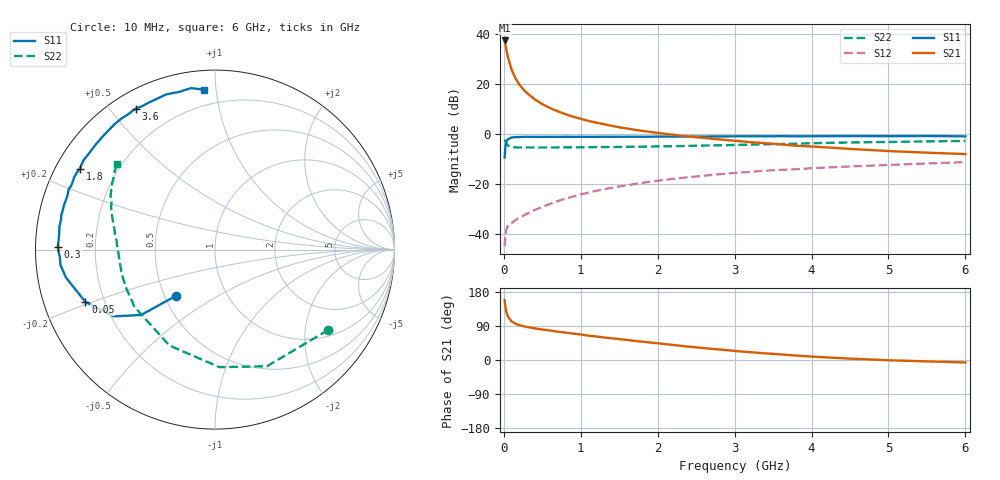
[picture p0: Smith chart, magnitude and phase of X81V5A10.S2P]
! SIEMENS Small Signal Semiconductors
! BFP136W
! Si NPN RF Bipolar Junction Transistor in SOT343
! VCE = 1.5 V  IC = 100 mA
! Common Emitter S-Parameters:  September  1994
# GHz  S  MA  R  50
!  f  S11  S21  S12  S22
! GHz  MAG  ANG  MAG  ANG  MAG  ANG  MAG  ANG
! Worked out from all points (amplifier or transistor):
!   40 points, 10 MHz to 6 GHz, reference 50 ohm
!   highest |S21| = 37.2 dB at 10 MHz (marker M1)
!   |S21| within 3 dB of that: start of sweep to 28.77 MHz
!   unconditionally stable (mu >= 1): 453.2 MHz to 2.977 GHz
!   at 200 MHz: K = 0.73, MSG = 26.5 dB, |S12| = -33.4 dB
!   at 1.5 GHz: K = 1.12, MAG = 9.7 dB, |S12| = -21.0 dB
!   at 6 GHz: K = 1.00, MSG = 1.6 dB, |S12| = -11.3 dB
!   S11 on the Smith chart (normalised r, x): 10 MHz: 0.57, -0.33; 50 MHz: 0.13, -0.19; 300 MHz: 0.07, +0.01; 1.8 GHz: 0.07, +0.28; 3.6 GHz: 0.07, +0.58; 6 GHz: 0.10, +0.93
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0.01  0.3386 -130.3  72.86 158.3  0.0058 66.9  0.7732 -35.4
0.02  0.5498 -138.5  61.04 140.9  0.0094 54.0  0.7114 -66.0
0.03  0.6754 -146.6  50.37 129.1  0.0121 47.2  0.6552 -87.9
0.05  0.7788 -158.0  35.11 115.5  0.0146 37.1  0.5917 -115.5
0.1  0.8451 -169.4  19.11 101.9  0.0168 35.9  0.5504 -144.6
0.15  0.8651 -174.3  12.94 95.9  0.0191 40.1  0.5391 -156.2
0.2  0.8655 -177.2  9.702 92.2  0.0215 42.8  0.5365 -162.3
0.25  0.8727 -179.6  7.821 89.4  0.0233 46.5  0.5366 -166.2
0.3  0.8767 179.0  6.533 87.3  0.0256 48.7  0.5348 -168.8
0.4  0.8725 175.8  4.922 83.5  0.0305 53.3  0.5358 -172.4
0.5  0.8735 173.2  3.924 80.3  0.0352 56.6  0.5364 -174.8
0.6  0.8765 171.4  3.275 77.8  0.0404 58.6  0.5372 -176.5
0.8  0.878 167.3  2.475 72.3  0.0513 61.3  0.5397 -179.0
1.1  0.8753 161.2  1.814 64.2  0.0677 61.9  0.5444 178.1
1.4  0.8766 156.2  1.45 57.3  0.0843 61.3  0.5485 175.7
1.8  0.8766 149.1  1.151 48.3  0.1059 58.6  0.5571 172.4
2.2  0.8834 142.6  0.962 39.7  0.1271 55.3  0.5691 169.2
3.2  0.8973 125.5  0.687 20.6  0.1753 45.4  0.6109 160.2
3.6  0.9018 119.4  0.619 14.8  0.1921 41.4  0.6298 156.6
4.5  0.9064 107.4  0.503 3.6  0.2252 32.7  0.676 148.5
5.5  0.9097 98.4  0.423 -3.7  0.2576 24.7  0.7106 141.8
6  0.8933 94.1  0.397 -6.4  0.2736 20.3  0.7235 138.9
